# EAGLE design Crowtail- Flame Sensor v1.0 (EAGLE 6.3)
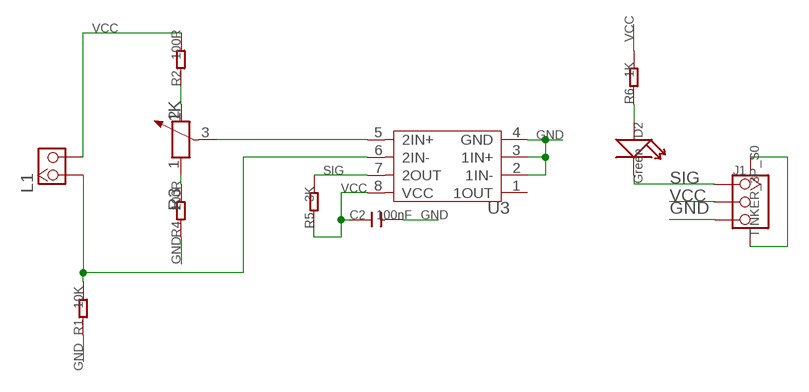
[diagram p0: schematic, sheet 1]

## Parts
C2  100nF  C-0603  [C0603]
D2  Green  LED'0603'  [LED-0603]
J1  TINKER_3P_S0  [TINKER_3P_S0]
L1  HEADER_1X2_2.54  [CK_1*2]
R1  10K  R-0603  [R0603]
R2  100R  R-0603  [R0603]
R3  1K  R-POTENTIOMETER'3362'  [3P-SQUA-7X6.8]
R4  100R  R-0603  [R0603]
R5  3K  R-0603  [R0603]
R6  1K  R-0603  [R0603]
U3  LM293D  [SOIC8-6.0]

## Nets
GND: C2.2 J1.3 J1.SS1 J1.SS2 R1.1 R4.1 U3.2(1IN-) U3.3(1IN+) U3.4(GND)
N$3: L1.1 R1.2 U3.6(2IN-)
N$4: R3.1 R4.2
N$5: R2.1 R3.2
N$6: R3.3 U3.5(2IN+)
N$7: D2.+ R6.1
SIG: D2.- J1.1 R5.2 U3.7(2OUT)
VCC: C2.1 J1.2 L1.2 R2.2 R5.1 R6.2 U3.8(VCC)
Unconnected: U3.1(1OUT)

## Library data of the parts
C2 = Discrete:C*: Ceramic Capacitors
D2 = Discrete:LED*
J1 = Connector:TINKER_3P_S0
L1 = CONNECTER:HEADER_1X2
R1 R2 R4-R6 = Discrete:R*
R3 = Discrete:R-POTENTIOMETER*: Potentiometer
U3 = IC:LM293: Dual Differential Comparator

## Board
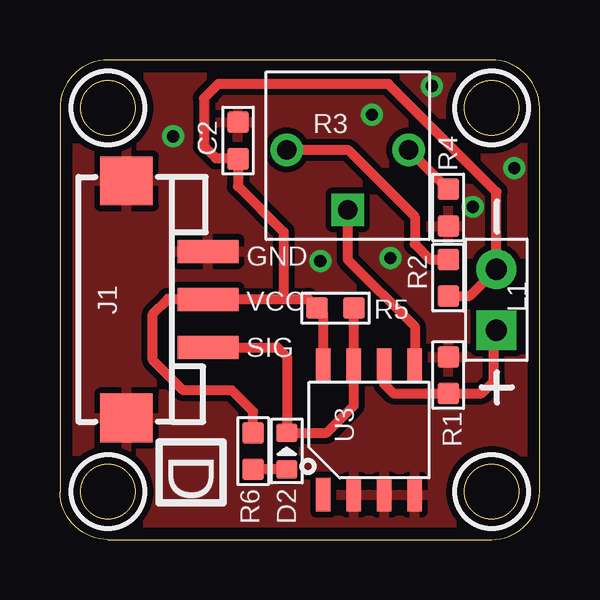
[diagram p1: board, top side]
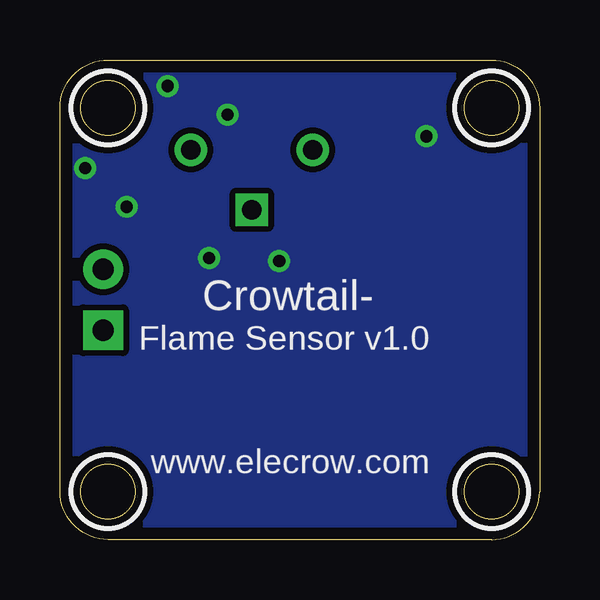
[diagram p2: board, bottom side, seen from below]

Size 20 x 20 mm. Coordinates in mm from the lower left corner, seen from the top.
Outline: 2,0 18,0 arc90 20,2 20,18 arc90 18,20 2,20 arc90 0,18 0,2 arc90 2,0
Outline: circle at 2,2 radius 1.14
Outline: circle at 18,2 radius 1.14
Outline: circle at 2,18 radius 1.14
Outline: circle at 18,18 radius 1.14
Copper layers (1*16): Top 0.035mm / dielectric 1.5mm / Bottom 0.035mm
Design rules "default *": minimum track width 10mil, minimum drill 20mil, track to track 8mil, track to pad 8mil, pad to pad 8mil, via to via 8mil, smd to smd 8mil, copper to edge 20mil, drill to drill 8mil, minimum pad ring 10mil, minimum via ring 8mil, stop-mask expansion 4mil, vias tented up to drill 100mil, thermal gap 10mil
tRestrict: area 0.5,0.5 to 3.5,3.5; area 16.5,0.5 to 19.5,3.5; area 0.5,16.5 to 3.5,19.5; area 16.5,16.5 to 19.5,19.5
bRestrict: area 0.5,0.5 to 3.5,3.5; area 16.5,0.5 to 19.5,3.5; area 0.5,16.5 to 3.5,19.5; area 16.5,16.5 to 19.5,19.5

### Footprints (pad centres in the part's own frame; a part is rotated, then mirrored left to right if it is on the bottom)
C0603 = smd 0.889 x 0.889: 1 -0.762,0; 2 0.762,0
LED-0603 = smd 0.762 x 0.889: + -0.762,0; - 0.762,0
TINKER_3P_S0 = smd 0.965 x 2.54: 1 -1.984,-3.175; 2 0.016,-3.175; 3 2.016,-3.175 | smd 2.032 x 2.184: SS1 -4.93,0.225; SS2 4.962,0.225
CK_1*2 = drill 0.889 pad 1.651 square: 1 0,1.27 | drill 0.889 pad 1.651: 2 0,-1.27
R0603 = smd 0.889 x 0.889: 1 -0.762,0; 2 0.762,0
3P-SQUA-7X6.8 = drill 0.8 pad 1.35: 1 -2.54,-0.25; 2 2.54,-0.25 | drill 0.8 pad 1.35 square: 3 0,2.25
SOIC8-6.0 = smd 0.6 x 1.4: 1 -1.905,-2.7; 2 -0.635,-2.7; 3 0.635,-2.7; 4 1.905,-2.7; 5 1.905,2.7; 6 0.635,2.7; 7 -0.635,2.7; 8 -1.905,2.7

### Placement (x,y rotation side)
C2  7.43,16.64 90 top
D2  9.46,3.69 90 top
J1  3,10 90 top
L1  18.2,10 180 top
R1  16.19,6.86 270 top
R2  16.19,10.92 270 top
R3  12,16 180 top
R4  16.19,13.84 90 top
R5  11.49,9.65 0 top
R6  8.06,3.69 90 top
U3  12.89,4.57 0 top

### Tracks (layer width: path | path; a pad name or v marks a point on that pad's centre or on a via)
GND  (via drill 0.51 pad 0.41)
  other vias: 13.02,17.71 13.78,11.74 10.86,11.62 15.52,18.91 4.71,16.81 17.21,13.88 18.94,15.48
  pour Bottom (isolate 0.254): 20.76,-0.51 20.89,20.45 -0.32,20.32 -0.45,-0.64
  pour Top (isolate 0.254): 20.89,-0.51 20.89,20.45 -0.45,20.32 -0.45,-0.64
N$3
  Top 0.406: L1.1 18.09,8.62 18.09,6.6 17.59,6.1 R1.2 13.9,6.1 13.52,6.48 U3.6
N$4
  Top 0.406: R4.2 R3.1
N$5
  Top 0.406: R3.2 12,16.25 14.79,13.46 14.79,12.32 15.43,11.68 R2.1
N$6
  Top 0.406: R3.3 12,11.68 14.79,8.89 U3.5
N$7
  Top 0.406: D2.+ R6.1
SIG
  Top 0.406: R5.2 U3.7 12.25,5.59 11.12,4.45 D2.- 9.46,7.62 9.06,8.02 J1.1
VCC
  Top 0.406: U3.8 10.98,9.4 R5.1 10.35,10.03 9.33,10.03 | R6.2 8.06,5.33 7.17,6.22 5.14,6.22 3.87,7.49 3.87,9.4 4.51,10.03 6.16,10.03 | 6.16,10.03 J1.2 | 6.16,10.03 9.33,10.03 | 9.33,10.03 9.33,12.83 7.43,14.73 C2.1 7.4,15.9 6.5,15.9 6,16.4 6,18.4 6.6,19 13.7,19 18.2,14.5 L1.2 17.09,10.16 R2.2

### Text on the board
tPlace: GND | VCC | SIG | D
bPlace: Crowtail- | Flame Sensor v1.0 | www.elecrow.com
